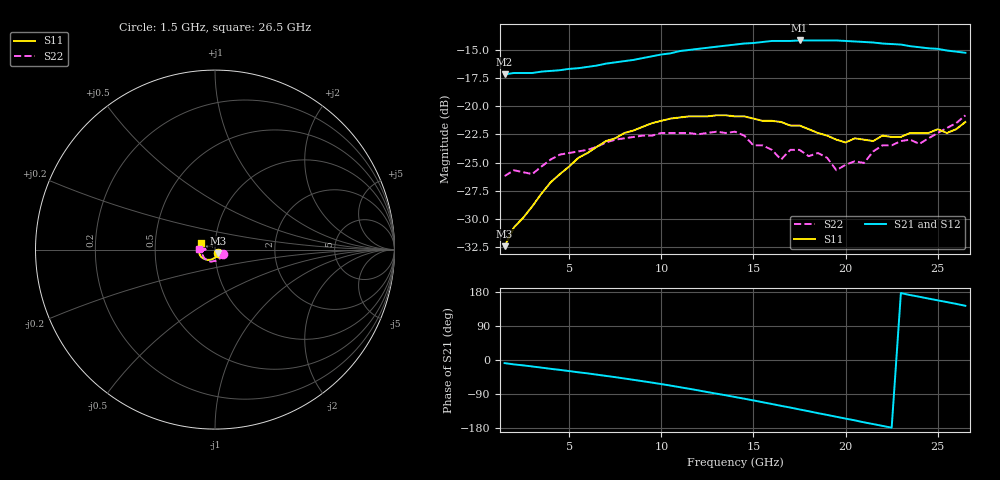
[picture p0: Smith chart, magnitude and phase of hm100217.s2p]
! HMMC-1002
! S-PARAMETERS at 17 dB attenuation setting. LAST UPDATED  07-06-99
# GHZ  S  MA  R  50
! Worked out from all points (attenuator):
!   51 points, 1.5 GHz to 26.5 GHz, reference 50 ohm
!   highest |S21| = -14.20 dB at 17.5 GHz (marker M1); lowest = -17.2 dB at 1.5 GHz (marker M2)
!   lowest |S11| = -32.4 dB at 1.5 GHz (marker M3), VSWR 1.05, Z = 51.5 - j1.9 ohm
!   |S11| at or under -10 dB: start of sweep to end of sweep
!   |S22| runs from -26.2 to -20.8 dB; largest |S21 - S12| = 0.0039
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1.5  0.024 -50.1  0.138 -8.3  0.138 -8.7  0.049 -26.5
2  0.029 -61.0  0.14 -11.5  0.14 -12.0  0.052 -34.6
3  0.036 -78.5  0.14 -17.1  0.14 -17.5  0.05 -51.9
4  0.046 -91.8  0.143 -23.3  0.143 -23.6  0.058 -65.1
6  0.062 -115.5  0.149 -35.3  0.149 -35.7  0.064 -94.1
10  0.086 -150.3  0.169 -63.5  0.169 -63.7  0.076 -136.3
14  0.09 -179.6  0.187 -97.7  0.187 -97.7  0.077 -170.5
16  0.086 169.9  0.194 -116.1  0.193 -116.1  0.064 178.6
16.5  0.085 165.9  0.194 -121.0  0.194 -120.8  0.058 178.3
17  0.082 164.2  0.194 -125.5  0.194 -125.5  0.064 179.4
17.5  0.082 163.3  0.195 -130.5  0.195 -130.4  0.064 175.0
18  0.079 160.8  0.195 -135.2  0.195 -135.0  0.06 177.6
18.5  0.076 161.1  0.195 -140.3  0.195 -139.9  0.062 -178.5
19.5  0.071 158.5  0.195 -149.8  0.194 -149.5  0.052 179.2
20.5  0.072 159.7  0.193 -159.3  0.193 -159.0  0.057 174.3
21  0.071 158.3  0.192 -164.5  0.191 -164.0  0.056 176.8
22  0.074 161.1  0.189 -173.9  0.189 -173.6  0.067 -177.6
22.5  0.073 158.7  0.188 -178.6  0.188 -178.4  0.067 -173.7
23.5  0.076 158.5  0.184 171.4  0.184 172.2  0.071 -174.9
24  0.076 155.1  0.182 166.9  0.182 167.5  0.068 179.9
25.5  0.076 153.8  0.176 152.8  0.176 153.0  0.08 176.1
26.5  0.085 155.0  0.172 143.0  0.172 144.3  0.091 177.5
